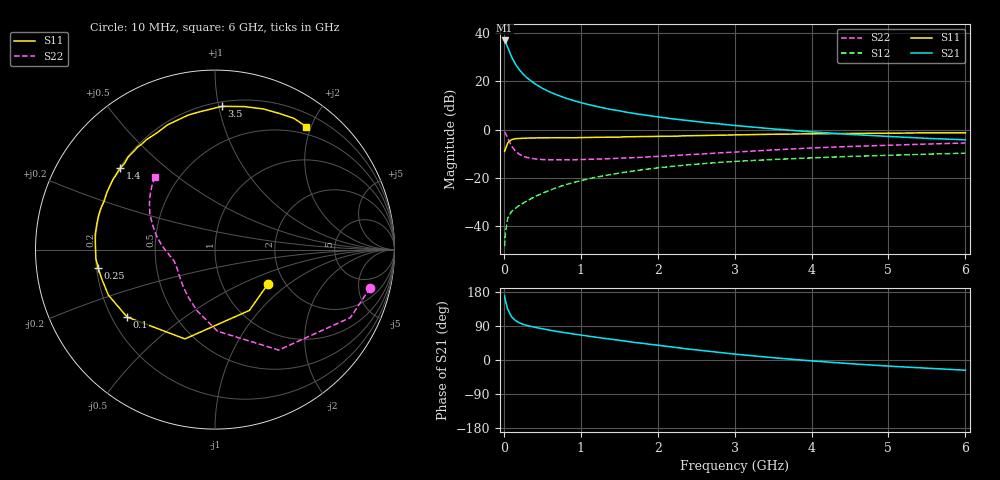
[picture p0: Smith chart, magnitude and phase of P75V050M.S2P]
! SIEMENS Small Signal Semiconductors
! BFP196
! Si NPN RF Bipolar Junction Transistor in SOT143
! VCE = 5 V  IC = 50 mA
! Common Emitter S-Parameters:  May  1996
# GHz  S  MA  R  50
!  f  S11  S21  S12  S22
! GHz  MAG  ANG  MAG  ANG  MAG  ANG  MAG  ANG
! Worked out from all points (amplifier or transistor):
!   36 points, 10 MHz to 6 GHz, reference 50 ohm
!   highest |S21| = 37.0 dB at 10 MHz (marker M1)
!   |S21| within 3 dB of that: start of sweep to 52.04 MHz
!   unconditionally stable (mu >= 1): 479.4 MHz to 4.423 GHz
!   at 250 MHz: K = 0.82, MSG = 26.8 dB, |S12| = -30.5 dB
!   at 1.4 GHz: K = 1.09, MAG = 11.7 dB, |S12| = -18.6 dB
!   at 6 GHz: K = 0.98, MSG = 2.8 dB, |S12| = -9.8 dB
!   S11 on the Smith chart (normalised r, x): 10 MHz: 1.64, -0.72; 100 MHz: 0.26, -0.32; 250 MHz: 0.21, -0.07; 1.4 GHz: 0.20, +0.36; 3.5 GHz: 0.23, +1.02; 6 GHz: 0.38, +1.93
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0.01  0.3518 -33.3  70.46 168.7  0.0038 80.3  0.8903 -13.9
0.02  0.3893 -60.5  65.84 157.4  0.0072 72.7  0.8445 -26.6
0.05  0.525 -108.6  50.81 134.1  0.0145 57.9  0.663 -57.6
0.1  0.6172 -142.5  32.3 114.1  0.0199 48.4  0.4547 -88.3
0.15  0.6459 -156.9  22.85 104.3  0.0232 48.2  0.3558 -106.1
0.2  0.6517 -165.5  17.54 98.3  0.0265 50.6  0.3071 -118.3
0.25  0.6595 -171.3  14.11 94.3  0.0297 53.3  0.2784 -127.8
0.3  0.6653 -175.6  11.85 91.2  0.0329 55.6  0.2637 -134.2
0.4  0.6672 177.5  8.974 86.5  0.0403 58.6  0.246 -144.0
0.5  0.6729 172.8  7.178 82.5  0.0476 61.0  0.2383 -150.5
0.6  0.6735 168.0  5.992 78.6  0.0554 61.4  0.2355 -154.8
0.7  0.6759 163.9  5.153 74.9  0.0632 61.8  0.2348 -158.2
0.9  0.674 156.2  4.014 68.9  0.0793 60.9  0.2354 -163.4
1.1  0.6844 149.0  3.3 62.9  0.0948 59.5  0.2412 -166.8
1.4  0.696 139.3  2.592 54.8  0.1171 56.1  0.2493 -171.0
1.7  0.7103 129.8  2.144 46.2  0.1389 52.3  0.2615 -175.4
2.2  0.7265 116.4  1.662 34.0  0.1728 45.0  0.2871 178.0
2.8  0.7643 101.2  1.31 20.1  0.2074 36.4  0.3273 168.4
3.5  0.7991 87.2  1.03 6.1  0.2389 26.5  0.377 157.9
4.5  0.8287 71.0  0.793 -9.7  0.2762 14.6  0.4447 145.2
5.5  0.8533 58.9  0.656 -21.6  0.3081 4.0  0.4998 134.7
6  0.8527 53.4  0.611 -27.0  0.323 -1.7  0.5254 129.6
